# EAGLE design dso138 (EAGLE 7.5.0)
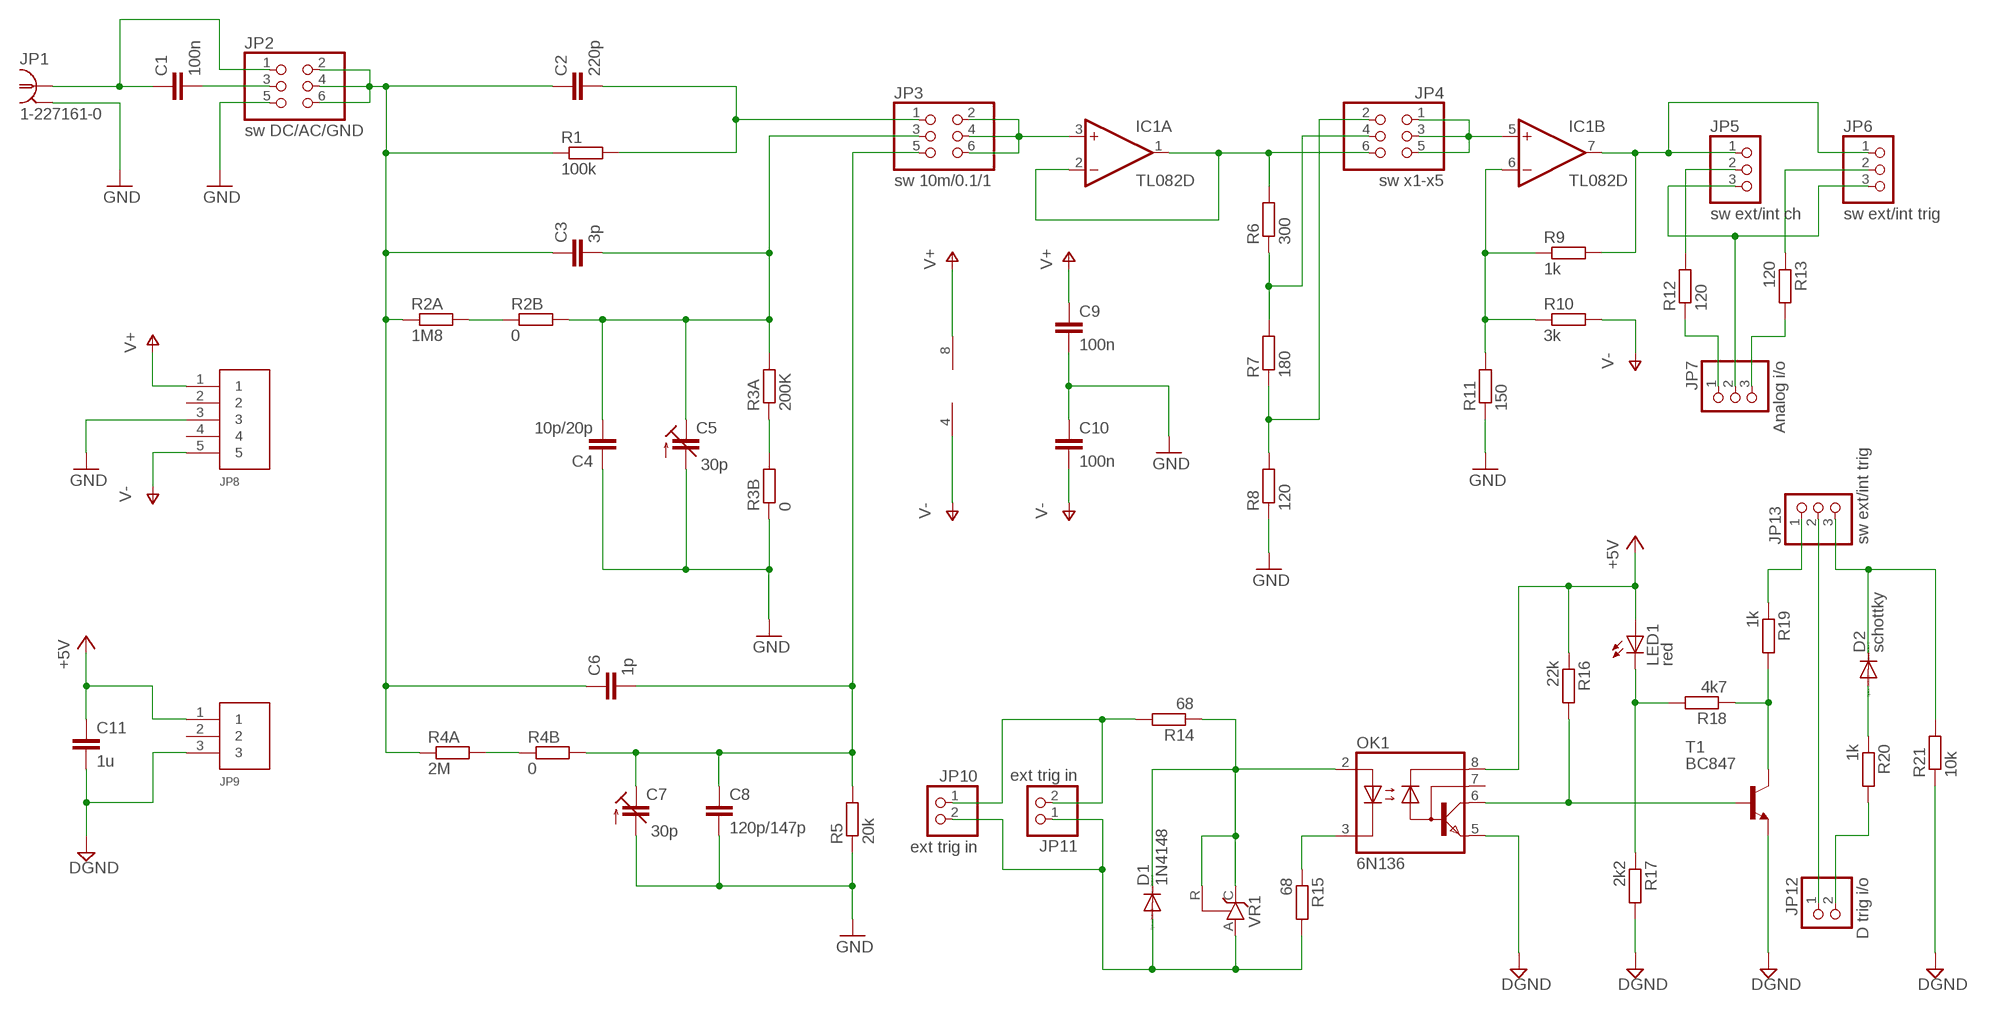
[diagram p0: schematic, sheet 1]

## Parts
C1  100n  C-EUC1206  [C1206]
C2  220p  C-EUC1206  [C1206]
C3  3p  C-EUC1206  [C1206]
C4  10p/20p  C-EUC1206  [C1206]
C5  30p  C-TRIMM3018_12  [CTRIM3018_12]
C6  1p  C-EUC1206  [C1206]
C7  30p  C-TRIMM3018_12  [CTRIM3018_12]
C8  120p/147p  C-EUC1206  [C1206]
C9  100n  C-EUC1206  [C1206]
C10  100n  C-EUC1206  [C1206]
C11  1u  C-EUC1206  [C1206]
D1  1N4148  DIODE-SOD80C  [SOD80C]
D2  schottky  DIODE-SOD80C  [SOD80C]
IC1  TL082D  [SO08]
JP1  1-227161-0  [AMP_227161]
JP2  sw DC/AC/GND  PINHD-2X3  [2X03]
JP3  sw 10m/0.1/1  PINHD-2X3  [2X03]
JP4  sw x1-x5  PINHD-2X3  [2X03]
JP5  sw ext/int ch  PINHD-1X3  [1X03]
JP6  sw ext/int trig  PINHD-1X3  [1X03]
JP7  Analog i/o  PINHD-1X3  [1X03]
JP8  PWR  5PIN  [B5B-PH-K-S]
JP9  3PIN  [B3B-PH-K-S]
JP10  ext trig in  PINHD-1X2  [1X02]
JP11  ext trig in  PINHD-1X2  [1X02]
JP12  D trig i/o  PINHD-1X2  [1X02]
JP13  sw ext/int trig  PINHD-1X3  [1X03]
LED1  red  LED3MM  [LED3MM]
OK1  6N136  CNW136  [DIL08HP4]
R1  100k  R-EU_R1206  [R1206]
R2A  1M8  R-EU_R1206  [R1206]
R2B  0  R-EU_R1206  [R1206]
R3A  200K  R-EU_R1206  [R1206]
R3B  0  R-EU_R1206  [R1206]
R4A  2M  R-EU_R1206  [R1206]
R4B  0  R-EU_R1206  [R1206]
R5  20k  R-EU_R1206  [R1206]
R6  300  R-EU_R1206  [R1206]
R7  180  R-EU_R1206  [R1206]
R8  120  R-EU_R1206  [R1206]
R9  1k  R-EU_R1206  [R1206]
R10  3k  R-EU_R1206  [R1206]
R11  150  R-EU_R1206  [R1206]
R12  120  R-EU_R1206  [R1206]
R13  120  R-EU_R1206  [R1206]
R14  68  R-EU_R1206  [R1206]
R15  68  R-EU_R1206  [R1206]
R16  22k  R-EU_R1206  [R1206]
R17  2k2  R-EU_R1206  [R1206]
R18  4k7  R-EU_R1206  [R1206]
R19  1k  R-EU_R1206  [R1206]
R20  1k  R-EU_R1206  [R1206]
R21  10k  R-EU_R1206  [R1206]
T1  BC847  [SOT23]
VR1  TL431CLP  [TO92-CLP]

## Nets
+5V: C11.1 JP9.1 LED1.A OK1.8(VCC) R16.1
DGND: C11.2 JP9.3 OK1.5(GND) R17.2 R21.1 T1.2(E)
GND: C4.1 C5.-(A) C7.-(A) C8.2 C9.2 C10.1 JP1.2 JP2.5 JP8.3 R3B.1 R5.1 R8.1 R11.1
N$1: IC1.3(A:+IN) JP3.2 JP3.4 JP3.6
N$2: C6.2 C7.+(E) C8.1 JP3.5 R4B.2 R5.2
N$3: C3.2 C4.2 C5.+(E) JP3.3 R2B.2 R3A.2
N$4: C2.2 JP3.1 R1.2
N$5: C2.1 C3.1 C6.1 JP2.2 JP2.4 JP2.6 R1.1 R2A.1 R4A.1
N$6: IC1.1(A:OUT) IC1.2(A:-IN) JP4.6 R6.2
N$7: JP4.4 R6.1 R7.2
N$8: JP4.2 R7.1 R8.2
N$9: IC1.6(B:-IN) R9.1 R10.1 R11.2
N$10: IC1.7(B:OUT) JP5.1 JP6.1 R9.2
N$11: C1.2 JP2.3
N$12: C1.1 JP1.1 JP2.1
N$13: IC1.5(B:+IN) JP4.1 JP4.3 JP4.5
N$14: R2A.2 R2B.1
N$15: R3A.1 R3B.2
N$16: R4A.2 R4B.1
N$17: D2.A R20.1
N$18: D2.C JP13.3 R21.2
N$19: D1.C OK1.2(A) R14.1 VR1.C VR1.R
N$20: D1.A JP10.2 JP11.1 R15.2 VR1.A
N$21: JP13.1 R19.1
N$22: LED1.K(C) R17.1 R18.2
N$23: OK1.3(C) R15.1
N$24: JP10.1 JP11.2 R14.2
N$25: R18.1 R19.2 T1.3(C)
N$26: JP5.3 JP6.3 JP7.2
N$27: JP12.2 R20.2
N$28: JP12.1 JP13.2
N$31: JP7.1 R12.1
N$32: JP5.2 R12.2
N$33: JP7.3 R13.2
N$34: JP6.2 R13.1
N$35: OK1.6(VO) R16.2 T1.1(B)
V+: C9.1 IC1.8(P:V+) JP8.1
V-: C10.2 IC1.4(P:V-) JP8.5 R10.2
Unconnected: JP8.2 JP8.4 JP9.2 OK1.7(VB)

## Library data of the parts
C1-C4 C6 C8-C11 = rcl:C-EU: CAPACITOR, European symbol
C5 C7 = rcl:C-TRIMM: Trimm capacitor
D1 D2 = diode:DIODE-: DIODE
IC1 = linear:TL082: OP AMP Data sheet; DATA_SHEET: <a href="http://www.ti.com/lit/ds/symlink/tl084a.pdf"> Data sheet </a>
JP1 = con-coax:?227161*: JACK, RIGHT ANGLE, 50 OHM, PCB, BNC; MF: TYCO ELECTRONICS; MPN: 1-227161; OC_FARNELL: unknown; OC_NEWARK: 33B3200
JP2-JP4 = pinhead:PINHD-2X3: PIN HEADER
JP5-JP7 JP13 = pinhead:PINHD-1X3: PIN HEADER
JP8 = jst_eph:5PIN
JP9 = jst_eph:3PIN
JP10-JP12 = pinhead:PINHD-1X2: PIN HEADER
LED1 = led:LED: LED
OK1 = optocoupler:CNW136: HEWLETT PACKARD OPTO COUPLER; MF: AGILENT TECHNOLOGIES; MPN: HCNW136-000E; OC_FARNELL: 9994742; OC_NEWARK: 88H7743
R1 R2A R2B R3A R3B R4A R4B R5-R21 = rcl:R-EU_: RESISTOR, European symbol
T1 = transistor:BC847: NPN TRANSISTOR
VR1 = v-reg:TL431CLP: VOLTAGE REGULATOR

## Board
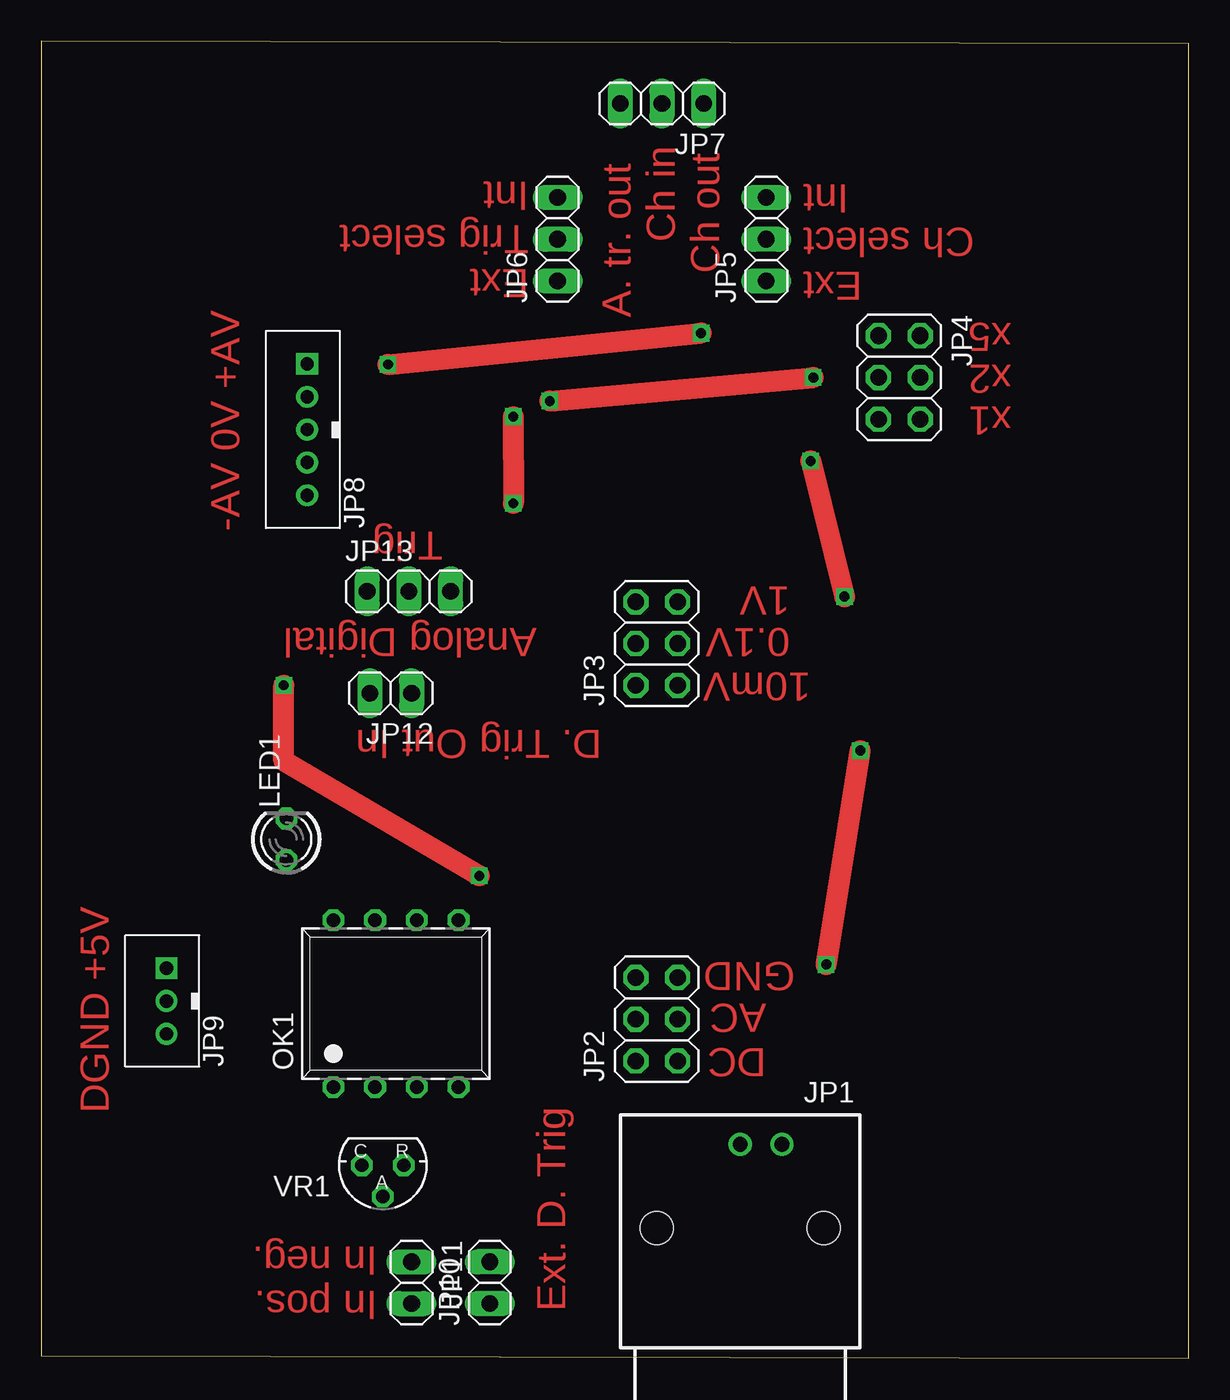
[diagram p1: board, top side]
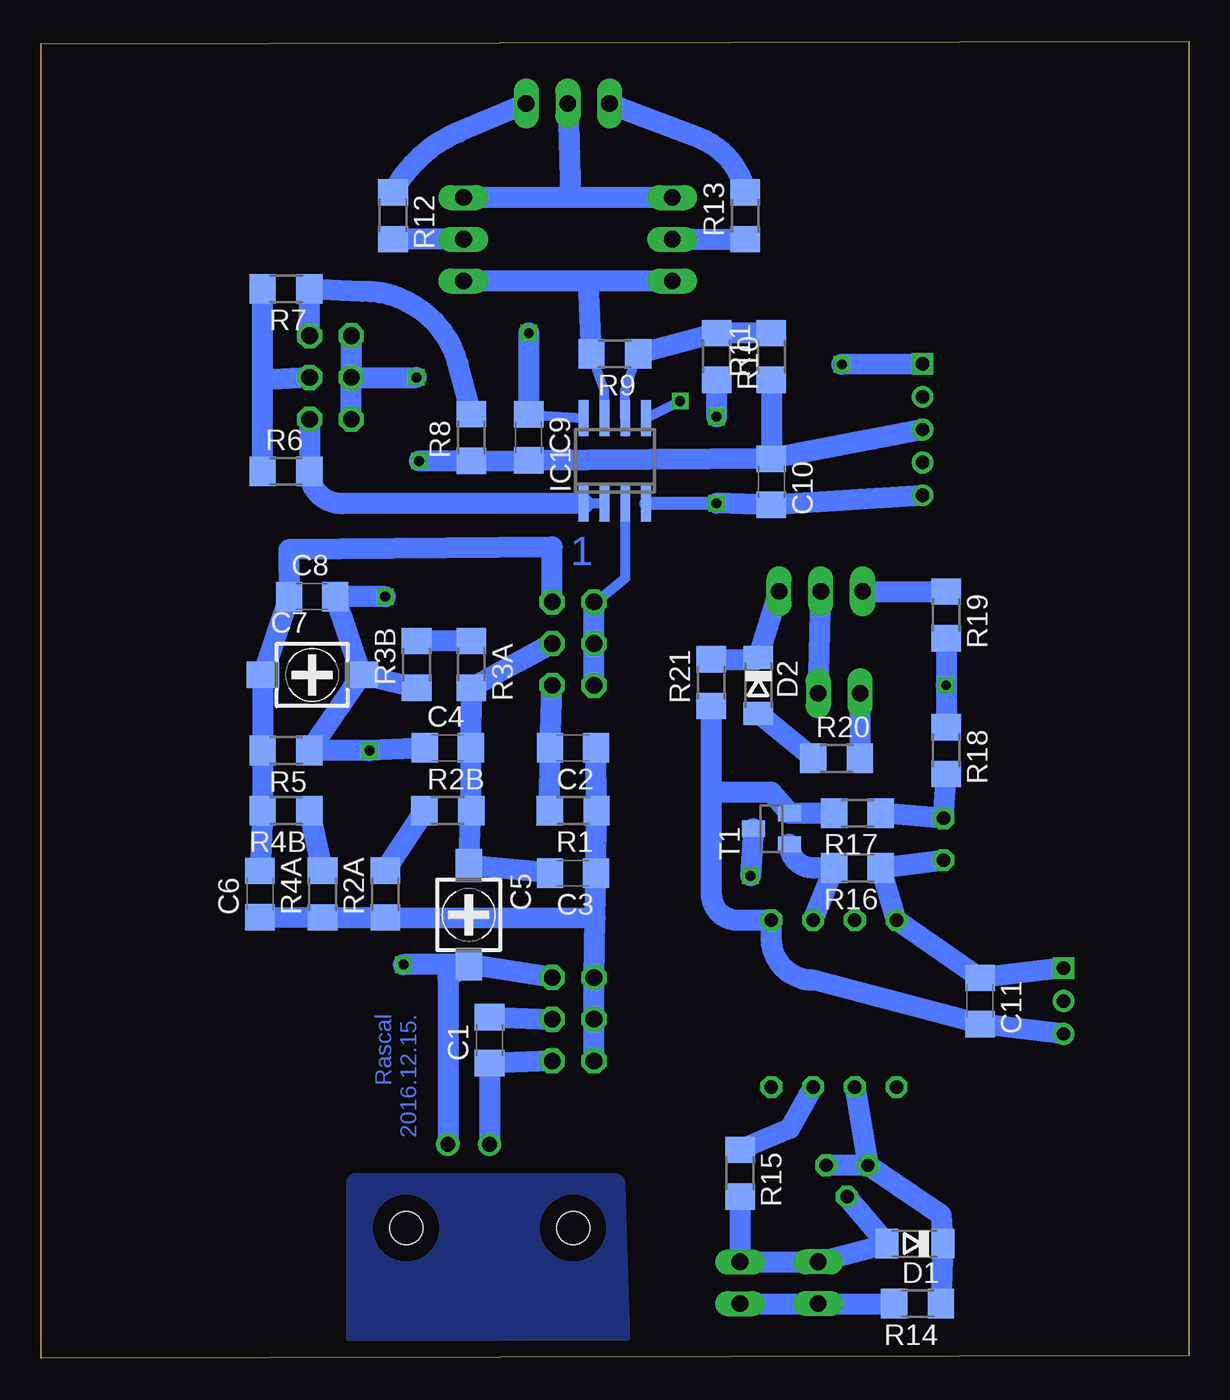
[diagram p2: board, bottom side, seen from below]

Size 69.84 x 80.16 mm. Coordinates in mm from the lower left corner, seen from the top.
Outline: 0,0.16 69.84,0 69.84,80 0,80.16 0,0.16
Copper layers (1*16): Top 0.035mm / dielectric 1.5mm / Bottom 0.035mm
Design rules "default": minimum track width 10mil, minimum drill 24mil, track to track 8mil, track to pad 8mil, pad to pad 8mil, via to via 8mil, smd to smd 8mil, copper to edge 40mil, drill to drill 8mil, minimum pad ring 10mil, minimum via ring 8mil, stop-mask expansion 4mil, vias tented up to drill 0mil, thermal gap 10mil

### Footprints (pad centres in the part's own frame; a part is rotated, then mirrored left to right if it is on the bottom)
C1206 = smd 1.6 x 1.8: 1 -1.4,0; 2 1.4,0
CTRIM3018_12 = smd 2 x 1.6: + -3,0; - 3,0
SOD80C = smd 1.4 x 1.8: A 1.7,0; C -1.7,0
SO08 = smd 0.6 x 2.2: 1 -1.905,-2.6; 2 -0.635,-2.6; 3 0.635,-2.6; 4 1.905,-2.6; 5 1.905,2.6; 6 0.635,2.6; 7 -0.635,2.6; 8 -1.905,2.6
AMP_227161 = drill 0.9 pad 1.27: 1 0,-5.08; 2 -2.54,-5.08 | hole 2: -5.08,0; 5.08,0
2X03 = drill 1.016 octagon: 1 -2.54,-1.27; 2 -2.54,1.27; 3 0,-1.27; 4 0,1.27; 5 2.54,-1.27; 6 2.54,1.27
1X03 = drill 1.016 long: 1 -2.54,0; 2 0,0; 3 2.54,0
B5B-PH-K-S = drill 0.813 square: 1 4,0 | drill 0.813: 2 2,0; 3 0,0; 4 -2,0; 5 -4,0
B3B-PH-K-S = drill 0.813 square: 1 2,0 | drill 0.813: 2 0,0; 3 -2,0
1X02 = drill 1.016 long: 1 -1.27,0; 2 1.27,0
LED3MM = drill 0.813 octagon: A -1.27,0; K 1.27,0
DIL08HP4 = drill 0.813 octagon: 1 -3.81,-5.08; 2 -1.27,-5.08; 3 1.27,-5.08; 4 3.81,-5.08; 5 3.81,5.08; 6 1.27,5.08; 7 -1.27,5.08; 8 -3.81,5.08
R1206 = smd 1.6 x 1.803: 1 -1.422,0; 2 1.422,0
SOT23 = smd 1 x 1.4: 1 -0.95,-1.1; 2 0.95,-1.1; 3 0,1.1
TO92-CLP = drill 0.813 octagon: A 0,1.905; C 1.27,0; R -1.27,0

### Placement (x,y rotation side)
C1  42.55,19.37 90 bottom
C2  37.47,37.15 180 bottom
C3  37.47,29.53 180 bottom
C4  45.09,37.15 0 bottom
C5  43.81,26.99 270 bottom
C6  56.52,28.26 90 bottom
C7  53.34,41.59 0 bottom
C8  53.34,46.35 0 bottom
C9  40.16,56.04 270 bottom
C10  25.4,53.34 270 bottom
C11  12.7,21.75 270 bottom
D1  16.67,6.99 180 bottom
D2  26.19,40.96 270 bottom
IC1  34.92,54.61 0 bottom
JP1  42.55,7.94 180 top
JP2  37.47,20.64 90 top
JP3  37.47,43.5 90 top
JP4  52.23,59.69 270 top
JP5  44.13,68.1 90 top
JP6  31.43,68.1 90 top
JP7  37.78,76.36 180 top
JP8  16.19,56.52 90 top
JP9  7.62,21.75 90 top
JP10  27.3,4.6 90 top
JP11  22.54,4.6 270 top
JP12  21.27,40.48 180 top
JP13  22.38,46.67 0 top
LED1  14.92,31.59 90 top
OK1  21.59,21.59 0 top
R1  37.47,33.34 180 bottom
R2A  48.9,28.26 90 bottom
R2B  45.09,33.34 0 bottom
R3A  43.66,42.23 270 bottom
R3B  46.99,42.23 90 bottom
R4A  52.7,28.26 90 bottom
R4B  54.93,33.34 180 bottom
R5  54.93,36.99 180 bottom
R6  54.93,53.97 0 bottom
R7  54.93,65.09 180 bottom
R8  43.66,56.04 90 bottom
R9  34.92,61.12 180 bottom
R10  28.73,60.96 270 bottom
R11  25.4,60.96 90 bottom
R12  48.42,69.53 270 bottom
R13  26.99,69.53 90 bottom
R14  16.51,3.33 180 bottom
R15  27.3,11.27 270 bottom
R16  20.16,29.85 180 bottom
R17  20.16,33.18 180 bottom
R18  14.76,36.99 270 bottom
R19  14.76,45.24 270 bottom
R20  21.43,36.51 0 bottom
R21  29.05,41.12 90 bottom
T1  25.4,32.23 90 bottom
VR1  20.8,11.75 180 top

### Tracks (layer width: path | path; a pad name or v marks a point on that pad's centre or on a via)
+5V
  Bottom 1.27: LED1.A R16.1 OK1.8 C11.1 JP9.1
DGND
  Bottom 1.27: JP9.3 C11.2 22.86,23.02 arc90 25.4,25.56 OK1.5 27.46,26.67 arc90 29.05,28.26 29.05,34.45 | 29.05,34.45 R21.1 | R17.2 T1.2 25.4,34.45 29.05,34.45
GND  (via drill 0.6)
  Top 1.27: v47.78,23.97 v49.85,36.99 | v46.83,54.61 v48.9,46.35
  Bottom 1.27: JP2.5 C5.- | C5.- 45.09,23.18 JP1.2 | C7.- R5.1 v49.85,36.99 C4.1 | C5.- v47.78,23.97 | C7.- C8.2 v48.9,46.35 | v46.83,54.61 R8.1 C9.2 C10.1 | R3B.1 C7.- | JP8.3 C10.1 | R11.1 C10.1
N$1
  Bottom 0.61: IC1.3 34.29,47.47 36.04,46.04 JP3.6
  Bottom 1.27: JP3.2 JP3.4 JP3.6
N$2
  Bottom 1.27: C6.2 R4B.2 R5.2 C7.+ C8.1 54.77,49.21 38.73,49.37 JP3.5
N$3
  Bottom 1.27: C3.2 C5.+ R2B.2 C4.2 R3A.2 40.8,42.39 JP3.3
N$4
  Bottom 1.27: R1.2 C2.2 JP3.1
N$5
  Bottom 1.27: JP2.2 JP2.4 JP2.6 36.12,26.82 | 36.12,26.82 C3.1 R1.1 C2.1 | C6.1 R4A.1 R2A.1 36.12,26.82
N$6
  Bottom 0.61: IC1.2 IC1.1
  Bottom 1.27: JP4.6 R6.2 arc-90 51.54,52.01 IC1.1
N$7
  Bottom 1.27: R6.1 56.35,59.53 | 56.35,59.53 R7.2 | JP4.4 56.35,59.53
N$8
  Bottom 1.27: R8.2 44.45,60.48 arc-76 50.32,64.93 R7.1 JP4.2
N$9
  Bottom 0.61: IC1.6 34.29,58.9 R9.1
  Bottom 1.27: R11.2 R10.1 R9.1
N$10
  Bottom 0.61: IC1.7 35.56,58.9 R9.2
  Bottom 1.27: JP6.1 36.51,65.56 | 36.51,65.56 JP5.1 | R9.2 36.51,65.56
N$11
  Bottom 1.27: C1.2 JP2.3
N$12
  Bottom 1.27: JP2.1 C1.1 JP1.1
N$13  (via drill 0.6)
  Top 1.27: v30.96,58.26 v46.99,59.69
  Bottom 0.61: IC1.5 v30.96,58.26
  Bottom 1.27: JP4.3 v46.99,59.69 | JP4.1 JP4.3 | JP4.5 JP4.3
N$14
  Bottom 1.27: R2B.1 R2A.2
N$15
  Bottom 1.27: R3A.1 R3B.2
N$16
  Bottom 1.27: R4A.2 R4B.1
N$17
  Bottom 1.27: R20.1 D2.A
N$18
  Bottom 1.27: R21.2 26.19,42.54 D2.C JP13.3
N$19
  Bottom 1.27: OK1.2 VR1.C | VR1.C VR1.R | VR1.C 15.08,8.73 D1.C R14.1
N$20
  Bottom 1.27: VR1.A D1.A JP11.1 JP10.2 R15.2
N$21
  Bottom 1.27: JP13.1 R19.1
N$22
  Bottom 1.27: R18.2 LED1.K R17.1
N$23
  Bottom 1.27: OK1.3 24.29,13.97 R15.1
N$24
  Bottom 1.27: JP10.1 JP11.2 R14.2
N$25  (via drill 0.6)
  Top 1.27: v26.67,29.37 14.76,36.35 v14.76,40.96
  Bottom 1.27: R19.2 v14.76,40.96 R18.1 | T1.3 v26.67,29.37
N$26
  Bottom 1.27: JP6.3 37.62,70.64 | 37.62,70.64 JP5.3 | JP7.2 37.62,70.64
N$27
  Bottom 1.27: JP12.2 R20.2
N$28
  Bottom 1.27: JP12.1 JP13.2
N$29
  pour Bottom: 34.92,10.64 50.64,10.64 50.64,1.11 34.61,1.11
N$31
  Bottom 1.27: JP7.1 44.45,74.61 arc-39 R12.1
N$32
  Bottom 1.27: JP5.2 R12.2
N$33
  Bottom 1.27: JP7.3 29.84,74.29 arc57 R13.2
N$34
  Bottom 1.27: JP6.2 R13.1
N$35
  Bottom 1.27: OK1.6 R16.2 22.87,29.84 arc90 T1.1
V+  (via drill 0.6)
  Top 1.27: v21.11,60.48 v40.16,62.39
  Bottom 0.61: C9.1 IC1.8
  Bottom 1.27: JP8.1 v21.11,60.48 | v40.16,62.39 C9.1
V-  (via drill 0.6)
  Top 1.27: v28.73,57.31 v28.74,52.03
  Bottom 0.813: v28.74,52.03 IC1.4
  Bottom 1.27: JP8.5 C10.2 v28.74,52.03 | R10.2 v28.73,57.31

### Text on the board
Top: Ext / Trig select / Int | Ext / Ch select / Int | Ch in | Ch out | A. tr. out | x5 | x2 | x1 | -AV 0V +AV | Trig | 1V | Analog Digital | 0.1V | 10mV | D. Trig Out In | GND | AC | DC | DGND +5V | In neg. | In pos. | Ext. D. Trig
Bottom: 1 | Rascal / 2016.12.15.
